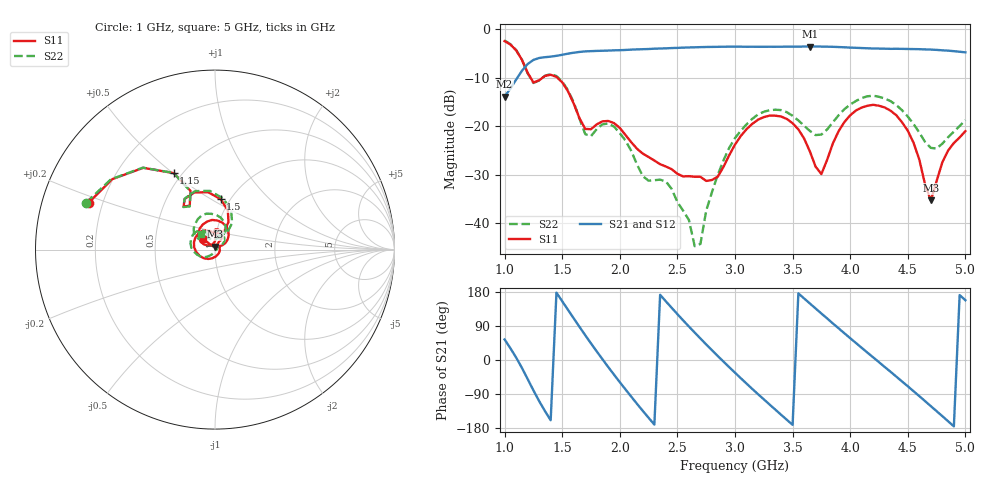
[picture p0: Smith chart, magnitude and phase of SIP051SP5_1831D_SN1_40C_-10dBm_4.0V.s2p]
# GHz  S  dB  R  50
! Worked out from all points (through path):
!   81 points, 1 GHz to 5 GHz, reference 50 ohm
!   highest |S21| = -3.59 dB at 3.65 GHz (marker M1); lowest = -13.9 dB at 1 GHz (marker M2)
!   lowest |S11| = -35.3 dB at 4.7 GHz (marker M3), VSWR 1.03, Z = 49.9 + j1.72 ohm
!   |S11| at or under -10 dB: 1.225 GHz to 1.331 GHz (105.4 MHz wide, 8.25 % of centre); 1.457 GHz to end of sweep
!   |S22| runs from -44.7 to -2.3 dB; largest |S21 - S12| = 0.0031
!   S11 on the Smith chart (normalised r, x): 1 GHz: 0.15, +0.18; 1.15 GHz: 0.45, +0.50; 1.5 GHz: 0.90, +0.55; 5 GHz: 0.87, +0.10
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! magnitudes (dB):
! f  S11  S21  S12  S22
! 1 GHz  -2.5  -13.9  -13.9  -2.3
! 1.15 GHz  -6.3  -8.6  -8.6  -6.3
! 1.25 GHz  -11.0  -6.3  -6.4  -11.1
! 1.5 GHz  -11.0  -5.3  -5.3  -10.8
! 1.7 GHz  -20.6  -4.6  -4.6  -21.6
! 1.95 GHz  -19.4  -4.4  -4.4  -20.1
! 2.2 GHz  -25.7  -4.1  -4.1  -30.3
! 2.35 GHz  -27.8  -4.0  -4.0  -31.0
! 2.65 GHz  -30.4  -3.7  -3.8  -44.7
! 2.7 GHz  -30.4  -3.7  -3.7  -44.2
! 2.8 GHz  -31.1  -3.7  -3.7  -33.6
! 3 GHz  -23.8  -3.6  -3.6  -22.4
! 3.35 GHz  -17.8  -3.6  -3.6  -16.6
! 3.65 GHz  -25.2  -3.6  -3.6  -21.0
! 3.7 GHz  -28.3  -3.6  -3.6  -21.8
! 3.75 GHz  -29.9  -3.6  -3.6  -21.7
! 4.05 GHz  -16.8  -3.9  -3.9  -14.8
! 4.35 GHz  -16.8  -4.1  -4.1  -14.8
! 4.55 GHz  -23.4  -4.1  -4.1  -19.5
! 4.7 GHz  -35.3  -4.2  -4.2  -24.5
! 4.85 GHz  -25.0  -4.4  -4.5  -22.3
! 5 GHz  -21.0  -4.8  -4.8  -18.7
